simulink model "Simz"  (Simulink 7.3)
settings: Solver=ode5  StartTime=0.0  StopTime=60  FixedStep=Ts  RelTol=1e-3
InitFcn:
  | r2d= 180/pi; d2r=1/r2d; Ts=0.04;                  % Radian to degree converts
  | [Azpl,Bzpl,Czpl,Dzpl]= plant_z;                   % Load Plant (Vehi,Actuat,Sensors)
  | [Apfc,Bpfc,Cpfc,Dpfc]= pitch_fcs;                 % Load Pitch FCS
  | [Alfc,Blfc,Clfc,Dlfc]= lateral_fcs;               % Load Lateral FCS
  | load TVC.Mat -ascii                               % Shuttle Stage-1 TVC Matrix at Max-Q
StopFcn:
  | pl
undefined symbols (not defined in the file or in its folder): Alfc, Apfc, Azpl, Blfc, Bpfc, Bzpl, Clfc, Cpfc, Czpl, Dlfc, Dpfc, Dzpl, TVC

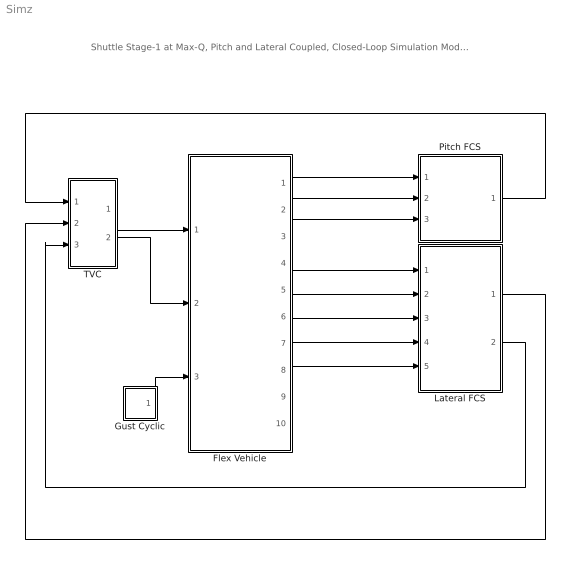
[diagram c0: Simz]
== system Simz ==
  note: Shuttle Stage-1 at Max-Q, Pitch and Lateral Coupled, Closed-Loop Simulation Model
  Flex Vehicle : Subsystem
  Gust Cyclic : Subsystem
  Lateral FCS : Subsystem
  Pitch FCS : Subsystem
  TVC : Subsystem
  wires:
  Pitch FCS/1(DQ_TVC) -> TVC/1(ptch)
  Lateral FCS/1(DP_TVC) -> TVC/2(roll)
  Lateral FCS/2(DR_TVC) -> TVC/3(yaw)
  TVC/2(dz) -> Flex Vehicle/2(dzc)
  TVC/1(dy) -> Flex Vehicle/1(dyc)
  Flex Vehicle/1(theta) -> Pitch FCS/1(theta)
  Flex Vehicle/2(q-flx) -> Pitch FCS/2(q)
  Flex Vehicle/3(Nz) -> Pitch FCS/3(Nz)
  Flex Vehicle/4(phi) -> Lateral FCS/1(phi-er)
  Flex Vehicle/5(psi) -> Lateral FCS/2(psi-er)
  Flex Vehicle/6(p-flx) -> Lateral FCS/3(p)
  Flex Vehicle/7(r-flx) -> Lateral FCS/4(r)
  Flex Vehicle/8(Ny) -> Lateral FCS/5(Ny)
  Gust Cyclic/1(Gust) -> Flex Vehicle/3(WG)

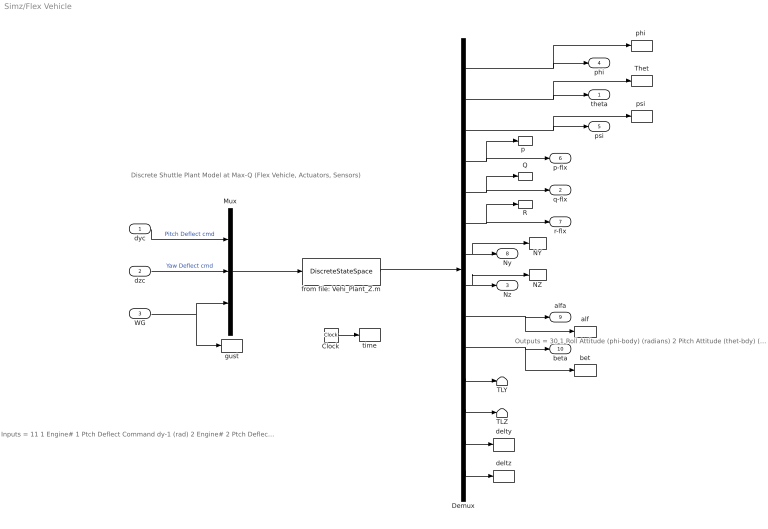
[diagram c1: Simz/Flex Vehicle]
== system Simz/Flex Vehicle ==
  note: Outputs = 30 1 Roll Attitude (phi-body) (radians) 2 Pitch Attitude (thet-bdy) (radians) 3 Yaw Attitude (psi-body) (radians) 4 Roll Rate Gyro (p-flex) (rad/sec) 5 Pitch Rate Gyro (q-flex) (rad/sec) 6 Yaw Rate Gyro (r-flex) (rad/sec) 7 Accelerom # 1, Y-ddot Accelerat. (ft/sec^2) 8 Accelerom # 2, Z-ddot Accelerat. (ft/sec^2) 9 Angle of attack, alfa, (radians) 10 Angle of sideslip, beta, (radian) 11 Load-Torque Pitch TLY-Eng-1 12 Load-Torque Pitch TLY-Eng-2 13 Load-Torque Pitch TLY-Eng-3 14 Load-Torque Pitch TLY-Eng-4 15 Load-Torque Pitch TLY-Eng-5 16 Load-Torque Yaw TLZ-Eng-1 17 Load-Torque Yaw TLZ-Eng-2 18 Load-Torque Yaw TLZ-Eng-3 19 Load-Torque Yaw TLZ-Eng-4 20 Load-Torque Yaw TLZ-Eng-5 21 Engine # 1 Pitch Deflection dy-1 (rad) 22 Engine # 2 Pitch Deflection dy-2 (rad) 23 Engine # 3 Pitch Deflection dy-3 (rad) 24 Engine # 4 Pitch Deflection dy-4 (rad) 25 Engine # 5 Pitch Deflection dy-5 (rad) 26 Engine # 1 Yaw Deflection dz-1 (rad) 27 Engine # 2 Yaw Deflection dz-2 (rad) 28 Engine # 3 Yaw Deflection dz-3 (rad) 29 Engine # 4 Yaw Deflection dz-4 (rad) 30 Engine # 5 Yaw Deflection dz-5 (rad)
  note: Inputs = 11 1 Engine# 1 Ptch Deflect Command dy-1 (rad) 2 Engine# 2 Ptch Deflect Command dy-2 (rad) 3 Engine# 3 Ptch Deflect Command dy-3 (rad) 4 Engine# 4 Ptch Deflect Command dy-4 (rad) 5 Engine# 5 Ptch Deflect Command dy-5 (rad) 6 Engine# 1 Yaw Deflect Command dz-1 (rad) 7 Engine# 2 Yaw Deflect Command dz-2 (rad) 8 Engine# 3 Yaw Deflect Command dz-3 (rad) 9 Engine# 4 Yaw Deflect Command dz-4 (rad) 10 Engine# 5 Yaw Deflect Command dz-5 (rad) 11 Wind Gust Velocity (ft/sec)
  note: Discrete Shuttle Plant Model at Max-Q (Flex Vehicle, Actuators, Sensors)
  dyc : Inport  PortDimensions=5  OutDataType=sfix(16)  OutScaling=2^0
  dzc : Inport  Port=2  PortDimensions=5  OutDataType=sfix(16)  OutScaling=2^0
  WG : Inport  Port=3  OutDataType=sfix(16)  OutScaling=2^0
  Clock : Clock
  Demux : Demux  Outputs=[1,1,1,1,1,1,1,1,1,1, 5,5,5,5]
  Mux : Mux  Inputs="[5  5  1]"
  NY : ToWorkspace  VariableName=Ny  SampleTime=-1  SaveFormat=Array
  NZ : ToWorkspace  VariableName=Nz  SampleTime=-1  SaveFormat=Array
  Q : ToWorkspace  VariableName=q  SampleTime=-1  SaveFormat=Array
  R : ToWorkspace  VariableName=r  SampleTime=-1  SaveFormat=Array
  TLY : Terminator
  TLZ : Terminator
  Thet : ToWorkspace  VariableName=theta  SampleTime=-1  SaveFormat=Array
  alf : ToWorkspace  VariableName=alpha  SampleTime=-1  SaveFormat=Array
  bet : ToWorkspace  VariableName=beta  SampleTime=-1  SaveFormat=Array
  delty : ToWorkspace  VariableName=delty  SampleTime=-1  SaveFormat=Array
  deltz : ToWorkspace  VariableName=deltz  SampleTime=-1  SaveFormat=Array
  from file: Vehi_Plant_Z.m : DiscreteStateSpace  A=Azpl  B=Bzpl  C=Czpl  D=Dzpl  SampleTime=Ts
  gust : ToWorkspace  VariableName=Gust  SampleTime=-1  SaveFormat=Array
  "p  " : ToWorkspace  VariableName=p  SampleTime=-1  SaveFormat=Array
  "phi " : ToWorkspace  VariableName=phi  SampleTime=-1  SaveFormat=Array
  "psi " : ToWorkspace  VariableName=psi  SampleTime=-1  SaveFormat=Array
  time : ToWorkspace  VariableName=time  SampleTime=-1  SaveFormat=Array
  theta : Outport  OutDataType=sfix(16)  OutScaling=2^0
  q-flx : Outport  Port=2  OutDataType=sfix(16)  OutScaling=2^0
  Nz : Outport  Port=3  OutDataType=sfix(16)  OutScaling=2^0
  phi : Outport  Port=4  OutDataType=sfix(16)  OutScaling=2^0
  psi : Outport  Port=5  OutDataType=sfix(16)  OutScaling=2^0
  p-flx : Outport  Port=6  OutDataType=sfix(16)  OutScaling=2^0
  r-flx : Outport  Port=7  OutDataType=sfix(16)  OutScaling=2^0
  Ny : Outport  Port=8  OutDataType=sfix(16)  OutScaling=2^0
  alfa : Outport  Port=9  OutDataType=sfix(16)  OutScaling=2^0
  beta : Outport  Port=10  OutDataType=sfix(16)  OutScaling=2^0
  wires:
  dyc/1 -> Mux/1  "Pitch Deflect cmd"
  dzc/1 -> Mux/2  "Yaw Deflect cmd"
  WG/1 -> Mux/3, gust/1
  Mux/1 -> from file: Vehi_Plant_Z.m/1
  from file: Vehi_Plant_Z.m/1 -> Demux/1
  Demux/1 -> phi/1, "phi "/1
  Demux/2 -> theta/1, Thet/1
  Demux/3 -> psi/1, "psi "/1
  Demux/4 -> p-flx/1, "p  "/1
  Demux/5 -> q-flx/1, Q/1
  Demux/6 -> r-flx/1, R/1
  Demux/7 -> Ny/1, NY/1
  Demux/8 -> Nz/1, NZ/1
  Demux/9 -> alfa/1, alf/1
  Demux/10 -> beta/1, bet/1
  Demux/11 -> TLY/1
  Demux/12 -> TLZ/1
  Demux/14 -> deltz/1
  Demux/13 -> delty/1
  Clock/1 -> time/1

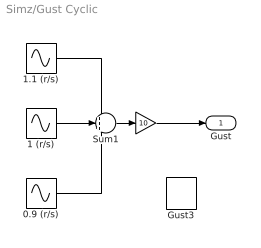
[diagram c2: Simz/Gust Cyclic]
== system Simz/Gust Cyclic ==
  " " : Gain  Gain=10  ParameterDataType=sfix(16)  ParameterScaling=2^0  OutDataType=sfix(16)  OutScaling=2^0
  0.9 (r/s) : Sin  Amplitude=1  Bias=0  Frequency=0.9  Phase=0  Samples=10  SampleTime=0
  1 (r/s) : Sin  Amplitude=1  Bias=0  Frequency=1  Phase=0  Samples=10  SampleTime=0
  1.1 (r/s) : Sin  Amplitude=1  Bias=0  Frequency=1.1  Phase=0  Samples=10  SampleTime=0
  Gust3 : DiscretePulseGenerator  PulseType=Time based  Amplitude=36  Period=100  PulseWidth=2  PhaseDelay=0  SampleTime=1
  Sum1 : Sum  Inputs=+++  OutDataType=fixdt(1, 16)  OutScaling=2^0
  Gust : Outport
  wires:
  Sum1/1 -> " "/1
  0.9 (r/s)/1 -> Sum1/3
  1 (r/s)/1 -> Sum1/2
  1.1 (r/s)/1 -> Sum1/1
  " "/1 -> Gust/1

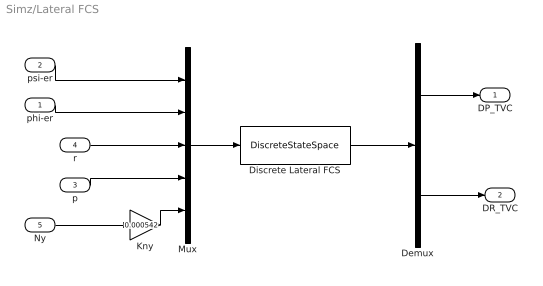
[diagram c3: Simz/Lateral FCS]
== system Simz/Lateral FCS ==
  phi-er : Inport  OutDataType=sfix(16)  OutScaling=2^0
  psi-er : Inport  Port=2  OutDataType=sfix(16)  OutScaling=2^0
  p : Inport  Port=3  OutDataType=sfix(16)  OutScaling=2^0
  r : Inport  Port=4  OutDataType=sfix(16)  OutScaling=2^0
  Ny : Inport  Port=5  OutDataType=sfix(16)  OutScaling=2^0
  Demux : Demux  Outputs=2
  Discrete Lateral FCS : DiscreteStateSpace  A=Alfc  B=Blfc  C=Clfc  D=Dlfc  SampleTime=Ts
  Kny : Gain  Gain=0.000542  ParameterDataType=sfix(16)  ParameterScaling=2^0  OutDataType=sfix(16)  OutScaling=2^0
  Mux : Mux  Inputs=5
  DP_TVC : Outport  OutDataType=sfix(16)  OutScaling=2^0
  DR_TVC : Outport  Port=2  OutDataType=sfix(16)  OutScaling=2^0
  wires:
  Kny/1 -> Mux/5
  Ny/1 -> Kny/1
  p/1 -> Mux/4
  Demux/2 -> DR_TVC/1
  Demux/1 -> DP_TVC/1
  Discrete Lateral FCS/1 -> Demux/1
  Mux/1 -> Discrete Lateral FCS/1
  r/1 -> Mux/3
  phi-er/1 -> Mux/2
  psi-er/1 -> Mux/1

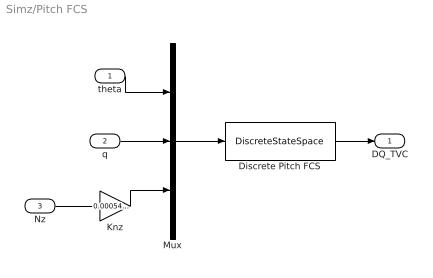
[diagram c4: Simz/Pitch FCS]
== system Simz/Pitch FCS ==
  theta : Inport  OutDataType=sfix(16)  OutScaling=2^0
  q : Inport  Port=2  OutDataType=sfix(16)  OutScaling=2^0
  Nz : Inport  Port=3  OutDataType=sfix(16)  OutScaling=2^0
  Discrete Pitch FCS : DiscreteStateSpace  A=Apfc  B=Bpfc  C=Cpfc  D=Dpfc  SampleTime=Ts
  Knz : Gain  Gain=0.000542*0.4  ParameterDataType=sfix(16)  ParameterScaling=2^0  OutDataType=sfix(16)  OutScaling=2^0
  Mux : Mux  Inputs=3
  DQ_TVC : Outport  OutDataType=sfix(16)  OutScaling=2^0
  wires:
  Knz/1 -> Mux/3
  Discrete Pitch FCS/1 -> DQ_TVC/1
  theta/1 -> Mux/1
  q/1 -> Mux/2
  Nz/1 -> Knz/1
  Mux/1 -> Discrete Pitch FCS/1

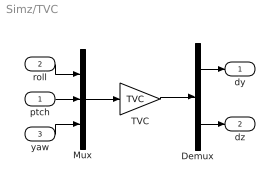
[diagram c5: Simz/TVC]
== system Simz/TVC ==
  ptch : Inport  OutDataType=sfix(16)  OutScaling=2^0
  roll : Inport  Port=2  OutDataType=sfix(16)  OutScaling=2^0
  yaw : Inport  Port=3  OutDataType=sfix(16)  OutScaling=2^0
  Demux : Demux  Outputs="[5  5]"
  Mux : Mux  Inputs=3
  TVC : Gain  Gain=TVC  Multiplication=Matrix(K*u) (u vector)  ParameterDataType=sfix(16)  ParameterScaling=2^0  OutDataType=sfix(16)  OutScaling=2^0
  dy : Outport  OutDataType=sfix(16)  OutScaling=2^0
  dz : Outport  Port=2  OutDataType=sfix(16)  OutScaling=2^0
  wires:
  TVC/1 -> Demux/1
  Mux/1 -> TVC/1
  roll/1 -> Mux/1
  Demux/1 -> dy/1
  ptch/1 -> Mux/2
  Demux/2 -> dz/1
  yaw/1 -> Mux/3
